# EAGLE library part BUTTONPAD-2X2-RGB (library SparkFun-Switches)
2x2 Button Pad w/ RGB LEDs Layout and schematic for 2x2 button pad with tri-color LEDs under each button. For use with the Button Pad 2x2 - LED Compatible and Button Pad 2x2 Top Bezel. Any RGB 5mm LED should be compatible. SparkFun Products SparkFun Simon Says - Through-Hole Soldering Kit (KIT-10547) Button Pad 2x2 - Breakout PCB (COM-09277)
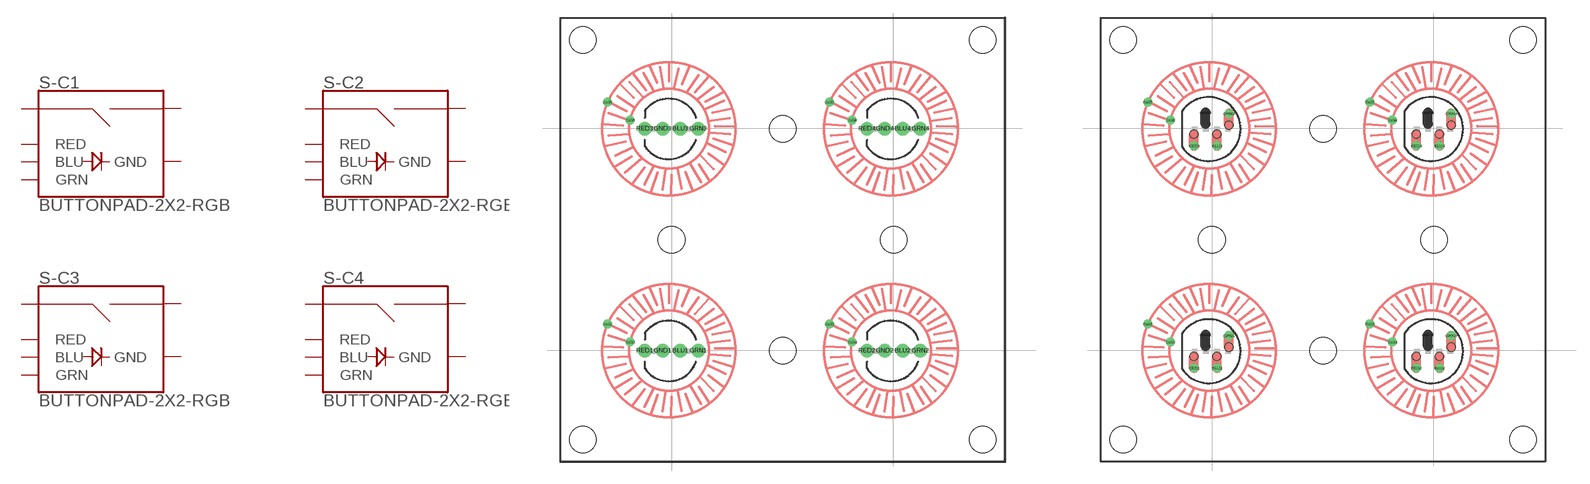
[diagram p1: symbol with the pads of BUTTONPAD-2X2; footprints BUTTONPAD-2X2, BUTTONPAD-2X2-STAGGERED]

Designator prefix S; gates -C1=BUTTONPAD-RGB -C2=BUTTONPAD-RGB -C3=BUTTONPAD-RGB -C4=BUTTONPAD-RGB

## BUTTONPAD-2X2-RGB (PROD_ID: COMP-08481; SF_SKU: COM-07836)  [BUTTONPAD-2X2]
BLU1  -C1:BLU
BLU2  -C2:BLU
BLU3  -C3:BLU
BLU4  -C4:BLU
GND1  -C1:GND
GND2  -C2:GND
GND3  -C3:GND
GND4  -C4:GND
GRN1  -C1:GRN
GRN2  -C2:GRN
GRN3  -C3:GRN
GRN4  -C4:GRN
RED1  -C1:RED
RED2  -C2:RED
RED3  -C3:RED
RED4  -C4:RED
SIG1  -C1:SIG1
SIG2  -C1:SIG2
SIG3  -C2:SIG1
SIG4  -C2:SIG2
SIG5  -C3:SIG1
SIG6  -C3:SIG2
SIG7  -C4:SIG1
SIG8  -C4:SIG2

## BUTTONPAD-2X2-RGB-STAGGERED (PROD_ID: COMP-08481; SF_SKU: COM-07836)  [BUTTONPAD-2X2-STAGGERED]
Pads as for BUTTONPAD-2X2

## Footprint BUTTONPAD-2X2 (pad centres in mm)
2x2 Button Pad w/ RGB LEDs Layout and schematic for 2x2 button pad with single-color LEDs under each button. For use with the Button Pad 2x2 - LED Compatible and Button Pad 2x2 Top Bezel. Any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
drill 1: BLU1 13.5,12.5; BLU2 38.5,12.5; BLU3 13.5,37.5; BLU4 38.5,37.5; GND1 11.5,12.5; GND2 36.5,12.5; GND3 11.5,37.5; GND4 36.5,37.5; GRN1 15.5,12.5; GRN2 40.5,12.5; GRN3 15.5,37.5; GRN4 40.5,37.5; RED1 9.5,12.5; RED2 34.5,12.5; RED3 9.5,37.5; RED4 34.5,37.5
drill 0.508: SIG1 5.288,15.513; SIG2 7.828,13.481; SIG3 30.288,15.513; SIG4 32.828,13.481; SIG5 5.288,40.513; SIG6 7.828,38.481; SIG7 30.288,40.513; SIG8 32.828,38.481
hole 3 at 12.5,25
hole 3 at 25,37.5
hole 3 at 37.5,25
hole 3 at 25,12.5
hole 3 at 2.5,2.5
hole 3 at 2.5,47.5
hole 3 at 47.5,47.5
hole 3 at 47.5,2.5

## Footprint BUTTONPAD-2X2-STAGGERED (pad centres in mm)
2x2 Button Pad w/ RGB LEDs - Staggered LED Footprint Layout and schematic for 2x2 button pad with single-color LEDs under each button. For use with the Button Pad 2x2 - LED Compatible and Button Pad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
drill 0.508: BLU1 13.081,10.566; BLU2 38.1,10.566; BLU3 13.081,35.585; BLU4 38.1,35.585; GND1 11.786,14.3; GND2 36.805,14.3; GND3 11.786,39.319; GND4 36.805,39.319; GRN1 14.427,14.199; GRN2 39.446,14.199; GRN3 14.427,39.218; GRN4 39.446,39.218; RED1 10.49,10.566; RED2 35.509,10.566; RED3 10.49,35.585; RED4 35.509,35.585; SIG1 5.288,15.513; SIG2 7.828,13.481; SIG3 30.288,15.513; SIG4 32.828,13.481; SIG5 5.288,40.513; SIG6 7.828,38.481; SIG7 30.288,40.513; SIG8 32.828,38.481
hole 3 at 12.5,25
hole 3 at 25,37.5
hole 3 at 37.5,25
hole 3 at 25,12.5
hole 3 at 2.5,2.5
hole 3 at 2.5,47.5
hole 3 at 47.5,47.5
hole 3 at 47.5,2.5
hole 0.914 at 10.49,36.881
hole 0.914 at 11.786,38.024
hole 0.914 at 13.081,36.881
hole 0.914 at 14.427,37.922
hole 0.914 at 35.509,36.881
hole 0.914 at 36.805,38.024
hole 0.914 at 38.1,36.881
hole 0.914 at 39.446,37.922
hole 0.914 at 10.49,11.862
hole 0.914 at 11.786,13.005
hole 0.914 at 13.081,11.862
hole 0.914 at 14.427,12.903
hole 0.914 at 35.509,11.862
hole 0.914 at 36.805,13.005
hole 0.914 at 38.1,11.862
hole 0.914 at 39.446,12.903

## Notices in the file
Licensing: Creative Commons ShareAlike 4.0 International - https://creativecommons.org/licenses/by-sa/4.0
